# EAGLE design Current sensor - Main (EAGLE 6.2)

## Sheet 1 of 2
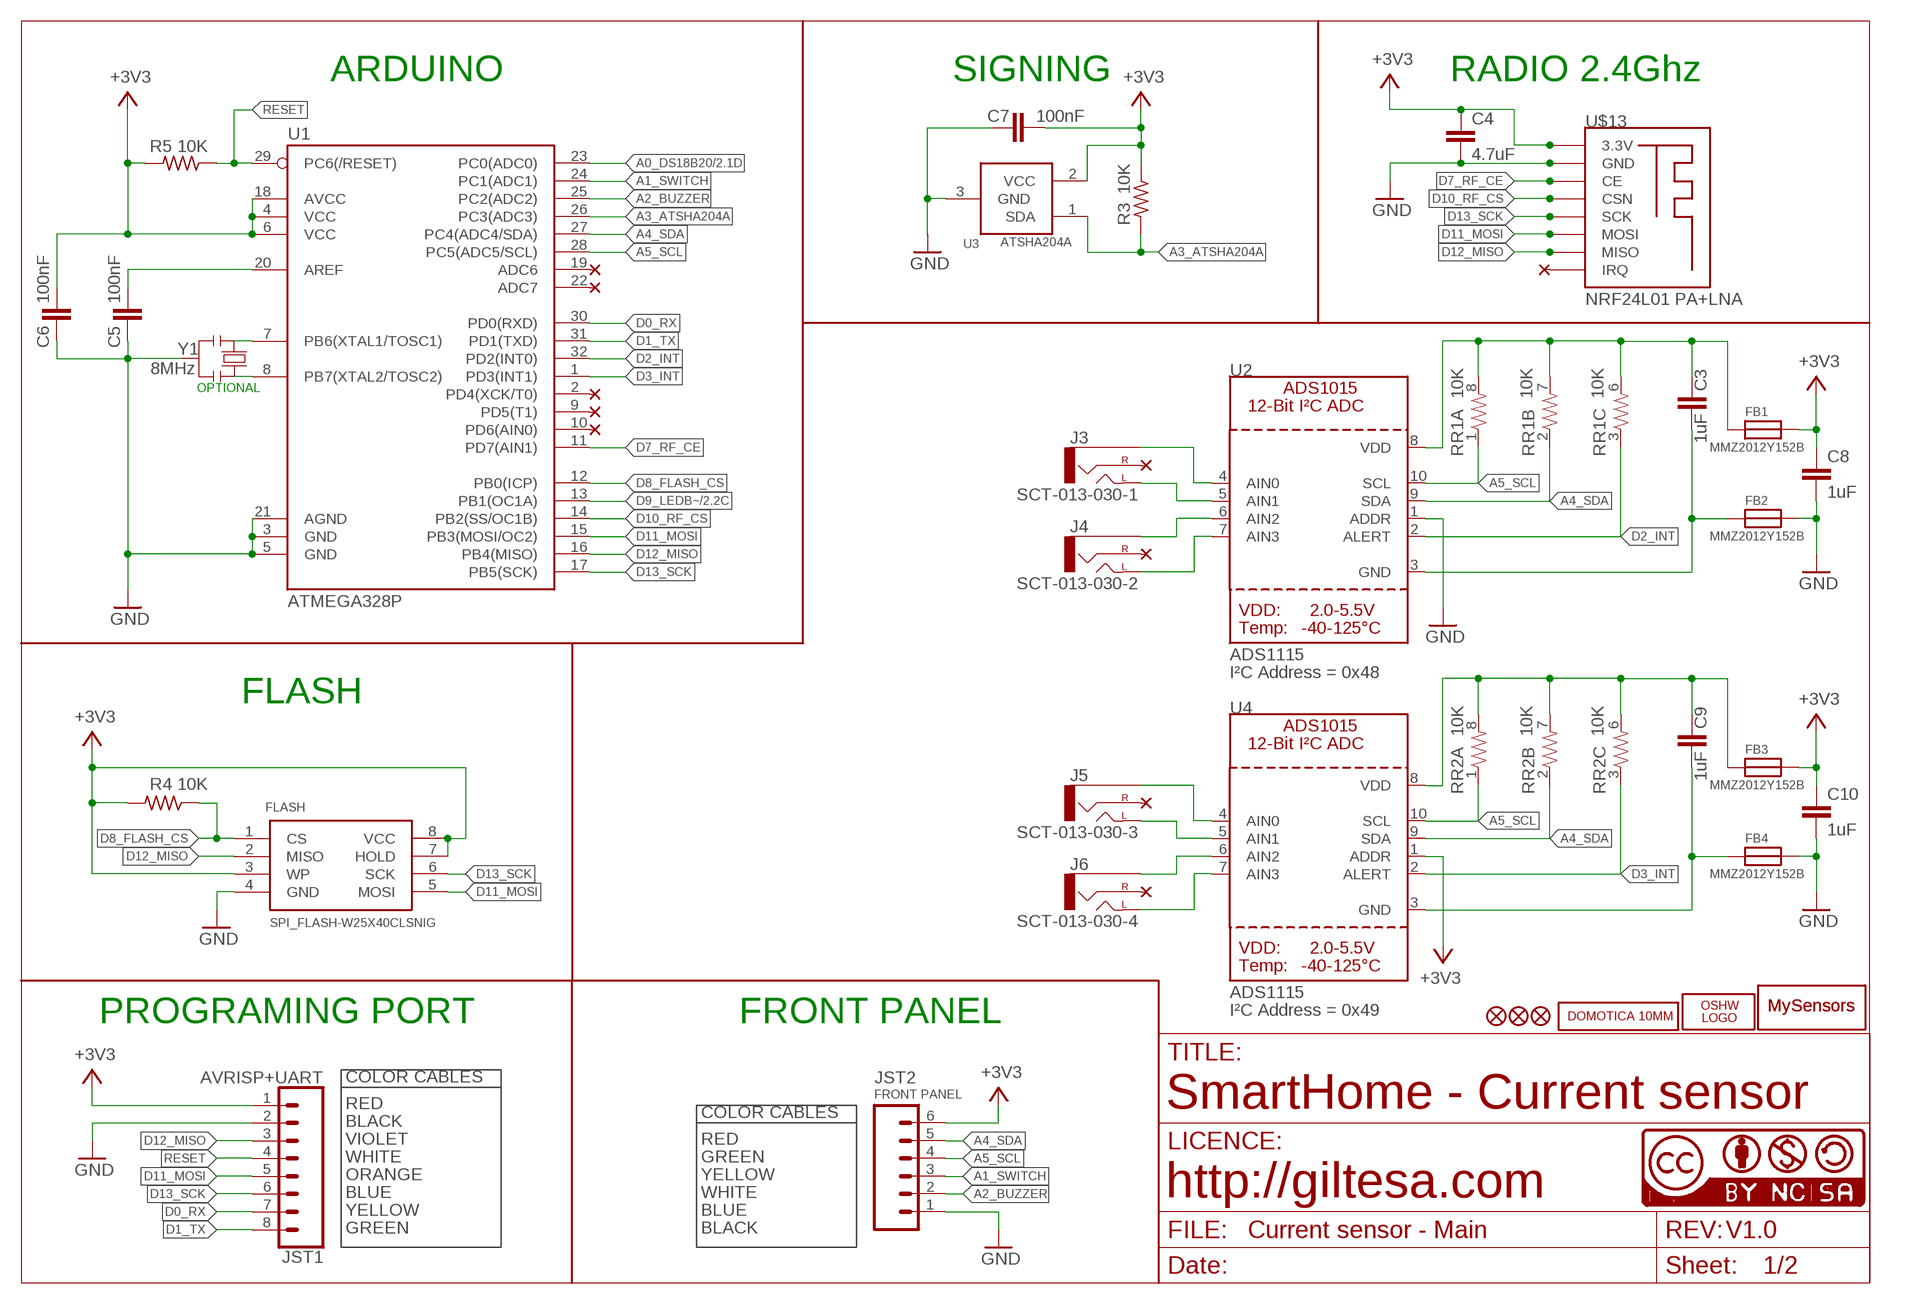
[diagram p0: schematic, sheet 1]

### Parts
C3  1uF  C0603  [C0603]
C4  4.7uF  C1206  [C1206]
C5  100nF  C0603  [C0603]
C6  100nF  C0603  [C0603]
C7  100nF  C0603  [C0603]
C8  1uF  C0603  [C0603]
C9  1uF  C0603  [C0603]
C10  1uF  C0603  [C0603]
FB1  MMZ2012Y152B  FERRITE0805  [0805]
FB2  MMZ2012Y152B  FERRITE0805  [0805]
FB3  MMZ2012Y152B  FERRITE0805  [0805]
FB4  MMZ2012Y152B  FERRITE0805  [0805]
FLASH  SPI_FLASH-W25X40CLSNIG  SPI_FLASH-X25XXSMD  [SO08]
J3  SCT-013-030-1  JACK_3.5MM  [JACK_3.5MM]
J4  SCT-013-030-2  JACK_3.5MM  [JACK_3.5MM]
J5  SCT-013-030-3  JACK_3.5MM  [JACK_3.5MM]
J6  SCT-013-030-4  JACK_3.5MM  [JACK_3.5MM]
JST1  AVRISP+UART  JST-8-1MM-SMD1  [JST-8-1MM-SMD]
JST2  FRONT PANEL  JST-6_1MM_SMD  [JST-6-1MM-SMD]
LOGO1  OSHW_LOGO_FILLX0150-NT  [OSHW_FILLX150_NOTEXT]
R3  10K  R0603  [R0603]
R4  10K  R0603  [R0603]
R5  10K  R0603  [R0603]
RR1  10K  RESISTOR-ARRAY0603-ARV  [0603-ARV]
RR2  10K  RESISTOR-ARRAY0603-ARV  [0603-ARV]
U1  ATMEGA328P  ATMEGA328P_TQFP  [TQFP32-08]
U2  ADS1115  ADC_ADS1015  [MSOP10]
U3  ATSHA204A  IC_ATSHA204A_CRYPT  [SOT23-3]
U4  ADS1115  ADC_ADS1015  [MSOP10]
U$2  MYSENSORS2  [MYSENSORS_20MM]
U$5  DOMOTICA-10MM  [DOMOTICA-10MM]
U$6  FIDUCIAL1X2  [FIDUCIAL-1X2]
U$7  FIDUCIAL1X2  [FIDUCIAL-1X2]
U$10  MYSENSORS4  [MYSENSORS_4MM]
U$13  NRF24L01 PA+LNA  NRF24L01SMD_RIGHT_IO2_B  [NRF24L01_SMD_RIGHT]
U$14  FIDUCIAL1X2  [FIDUCIAL-1X2]
U$20  CC-NC-BCNIX  [CC-NC-B_NIX]
Y1  8MHz  RESONATORMU  [RESONATOR]

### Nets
+3V3: C4.1 C6.2 C7.2 C8.1 C10.1 FB1.1 FB3.1 FLASH.3(WP) FLASH.7(HOLD) FLASH.8(VCC) JST1.1 JST2.6 R3.1 R4.2 R5.2 U1.4(VCC) U1.6(VCC) U1.18(AVCC) U3.2(VCC) U4.1(ADDR) U$13.B1(3.3V) ; also sheet 2
A0_DS18B20: U1.23(PC0(ADC0)) ; also sheet 2
A1_SWITCH: JST2.3 U1.24(PC1(ADC1))
A2_BUZZER: JST2.2 U1.25(PC2(ADC2))
A3_ATSHA204A: R3.2 U1.26(PC3(ADC3)) U3.1(SDA)
A4_SDA: JST2.5 RR1.2 RR2.2 U1.27(PC4(ADC4/SDA)) U2.9(SDA) U4.9(SDA)
A5_SCL: JST2.4 RR1.1 RR2.1 U1.28(PC5(ADC5/SCL)) U2.10(SCL) U4.10(SCL)
AIN0: J3.G U2.4(AIN0)
AIN1: J3.L U2.5(AIN1)
AIN2: J4.G U2.6(AIN2)
AIN3: J4.L U2.7(AIN3)
AIN4: J5.G U4.4(AIN0)
AIN5: J5.L U4.5(AIN1)
AIN6: J6.G U4.6(AIN2)
AIN7: J6.L U4.7(AIN3)
D0_RX: JST1.7 U1.30(PD0(RXD))
D1_TX: JST1.8 U1.31(PD1(TXD))
D2_INT: RR1.3 U1.32(PD2(INT0)) U2.2(ALERT)
D3_INT: RR2.3 U1.1(PD3(INT1)) U4.2(ALERT)
D7_RF_CE: U1.11(PD7(AIN1)) U$13.B2(CE)
D8_FLASH_CS: FLASH.1(CS) R4.1 U1.12(PB0(ICP))
D9_LEDB~: U1.13(PB1(OC1A)) ; also sheet 2
D10_RF_CS: U1.14(PB2(SS/OC1B)) U$13.B3(CSN)
D11_MOSI: FLASH.5(MOSI) JST1.5 U1.15(PB3(MOSI/OC2)) U$13.B5(MOSI)
D12_MISO: FLASH.2(MISO) JST1.3 U1.16(PB4(MISO)) U$13.B6(MISO)
D13_SCK: FLASH.6(SCK) JST1.6 U1.17(PB5(SCK)) U$13.B4(SCK)
GND: C4.2 C5.1 C6.1 C7.1 C8.2 C10.2 FB2.1 FB4.1 FLASH.4(GND) JST1.2 JST2.1 U1.3(GND) U1.5(GND) U1.21(AGND) U2.1(ADDR) U3.3(GND) U$13.B8(GND) Y1.2 ; also sheet 2
N$1: C9.2 FB3.2 RR2.6 RR2.7 RR2.8 U4.8(VDD)
N$2: C9.1 FB4.2 U4.3(GND)
N$3: C3.2 FB1.2 RR1.6 RR1.7 RR1.8 U2.8(VDD)
N$4: C3.1 FB2.2 U2.3(GND)
N$29: U1.7(PB6(XTAL1/TOSC1)) Y1.1
N$30: U1.8(PB7(XTAL2/TOSC2)) Y1.3
N$33: C5.2 U1.20(AREF)
RESET: JST1.4 R5.1 U1.29(PC6(/RESET))
Unconnected: J3.R J4.R J5.R J6.R RR1.4 RR1.5 RR2.4 RR2.5 U1.2(PD4(XCK/T0)) U1.9(PD5(T1)) U1.10(PD6(AIN0)) U1.19(ADC6) U1.22(ADC7) U$13.B7(IRQ)

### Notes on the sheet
- ARDUINO | SIGNING | RADIO 2.4Ghz
- OPTIONAL
- I²C Address = 0x48
- FLASH
- I²C Address = 0x49
- PROGRAMING PORT | FRONT PANEL
- COLOR CABLES
- RED | SmartHome - Current sensor
- COLOR CABLES
- BLACK
- VIOLET | RED
- WHITE | GREEN
- ORANGE | YELLOW
- BLUE | WHITE | http://giltesa.com
- YELLOW | BLUE
- GREEN | BLACK | V1.0

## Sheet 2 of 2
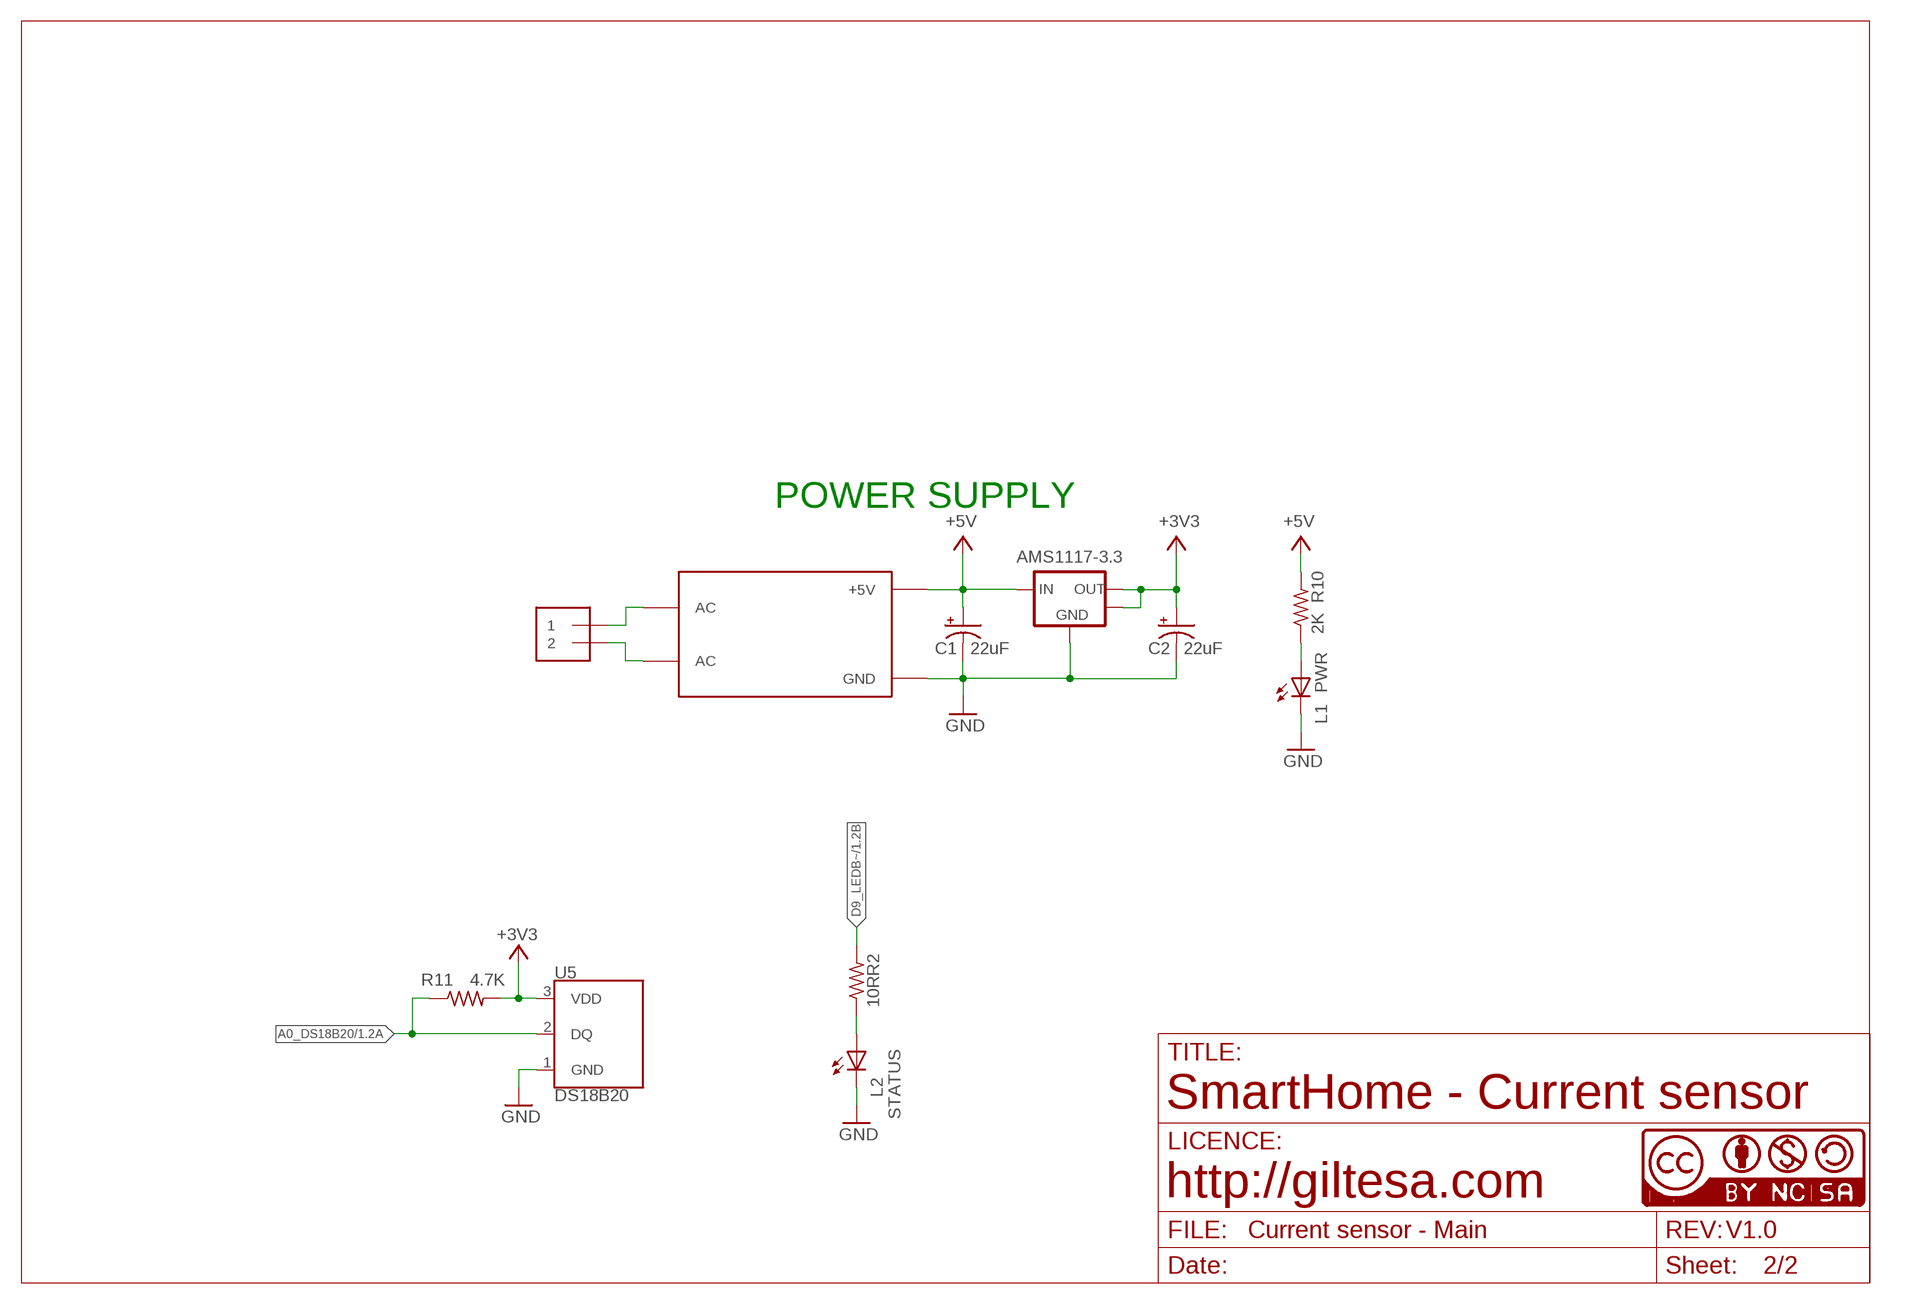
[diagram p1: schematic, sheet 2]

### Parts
AMS1117-3.3  AMS1117-3.3  AMS1117SOT89_2  [SOT89_2]
C1  22uF  CAP_POL3528  [EIA3528]
C2  22uF  CAP_POL3528  [EIA3528]
L1  PWR  LEDCHIP-LED0805  [CHIP-LED0805]
L2  STATUS  LEDCHIP-LED0805  [CHIP-LED0805]
R2  10R  R0603  [R0603]
R10  2K  R0603  [R0603]
R11  4.7K  R0603  [R0603]
U5  DS18B20  [DS18B20]
U$1  HILINK HLK-PM01 5V  HILINK_HLK-PM01_5V  [HILINK_HLK-PM01_5V]
U$12  230V  TERMINAL_15A_2PIN_RIGHT  [TERMINAL_15A_2PIN_RIGHT]
U$36  CC-NC-BCNIX  [CC-NC-B_NIX]

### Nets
+3V3: AMS1117-3.3.2(OUT) AMS1117-3.3.4(NC) C2.A(+) R11.2 U5.3(VDD) ; also sheet 1
+5V: AMS1117-3.3.3(IN) C1.A(+) R10.2 U$1.+5V
A0_DS18B20: R11.1 U5.2(DQ) ; also sheet 1
D9_LEDB~: R2.2 ; also sheet 1
GND: AMS1117-3.3.1(GND) C1.C(-) C2.C(-) L1.C L2.C U5.1(GND) U$1.GND ; also sheet 1
N$7: L2.A R2.1
N$8: L1.A R10.1
NEUTRAL: U$1.AC@2(AC) U$12.1
PHASE: U$1.AC@1(AC) U$12.2

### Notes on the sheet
- POWER SUPPLY
- SmartHome - Current sensor
- http://giltesa.com
- V1.0

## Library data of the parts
AMS1117-3.3 = ,giltesa:AMS1117
C1 C2 = SparkFun:CAP_POL: Capacitor Polarized
C3 C5-C10 = ,giltesa:C0603
C4 = ,giltesa:C1206
FB1-FB4 = microbuilder:FERRITE: Ferrite Bead
FLASH = SparkFun-DigitalIC:SPI_FLASH-X25XX: 8pin SPI Flash series x25xx. Works with devices like W25X32 and BR25L32
J3-J6 = ,giltesa:JACK_3.5MM
JST1 = ,giltesa:JST-8-1MM-SMD
JST2 = ,giltesa:JST-6
L1 L2 = led:LED: LED
LOGO1 = ohw-logo:OSHW_LOGO_FILL
R2-R5 R10 R11 = ,giltesa:R0603
RR1 RR2 = SparkFun-Passives:RESISTOR-ARRAY: Array Chip Resistor Source: RS Component / Phycomp
U1 = SparkFun-DigitalIC:ATMEGA328P_TQFP; PROD_ID: IC-09069; VALUE: ATMEGA328P_TQFP
U2 U4 = microbuilder:ADC_ADS1015: ADS1015 - 12-bit 4-Channel I2C ADC with Internal PGA VDD: 2.0-5.5V Sampling Rate: 3.3ksps Gain Settings: 2/3, 1, 2, 4, 8, 16 I2C Address: ADDR low = 1001000x, ADDR high = 1001001x Internal Comparator The ADS1015 includes an internal comparator that can be set to output a high-level on ALERT when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
U3 = TD-MySensors:IC_ATSHA204A_CRYPT
U5 = ,giltesa:DS18B20
U$1 = ,giltesa:HILINK_HLK-PM01_5V
U$2 U$10 = ,giltesa_logos:MYSENSORS
U$5 = ,giltesa_logos:DOMOTICA-10MM
U$6 U$7 U$14 = SparkFun:FIDUCIAL: Fiducial Alignment Points
U$12 = ,giltesa:TERMINAL_15A_2PIN_RIGHT
U$13 = ,giltesa:NRF24L01
U$20 U$36 = cc-by-nc-sa:CC-NC-BC: All hardware is licensed under the Creative Commons
Y1 = MySMD2:RESONATOR

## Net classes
2 gnd: width 0.305 mm, drill 0.406 mm, clearance 0.203 mm
3 usbvcc: width 0.203 mm, drill 0.406 mm, clearance 0.203 mm
4 USBpair: width 0.254 mm, drill 0.406 mm, clearance 0.61 mm

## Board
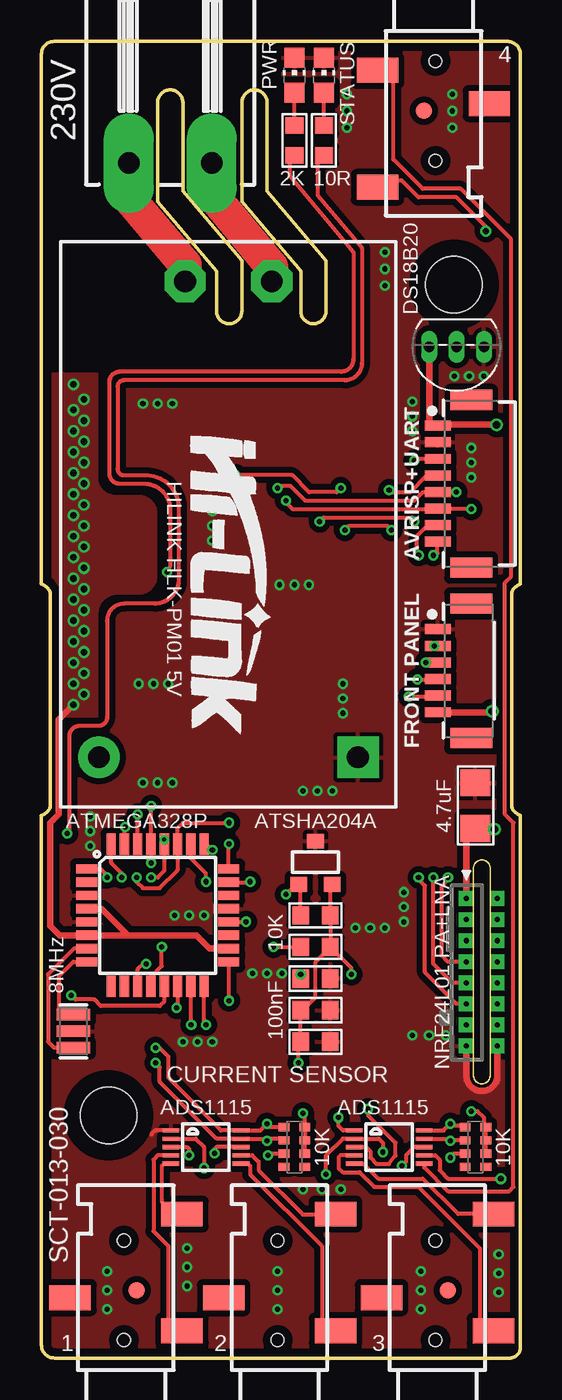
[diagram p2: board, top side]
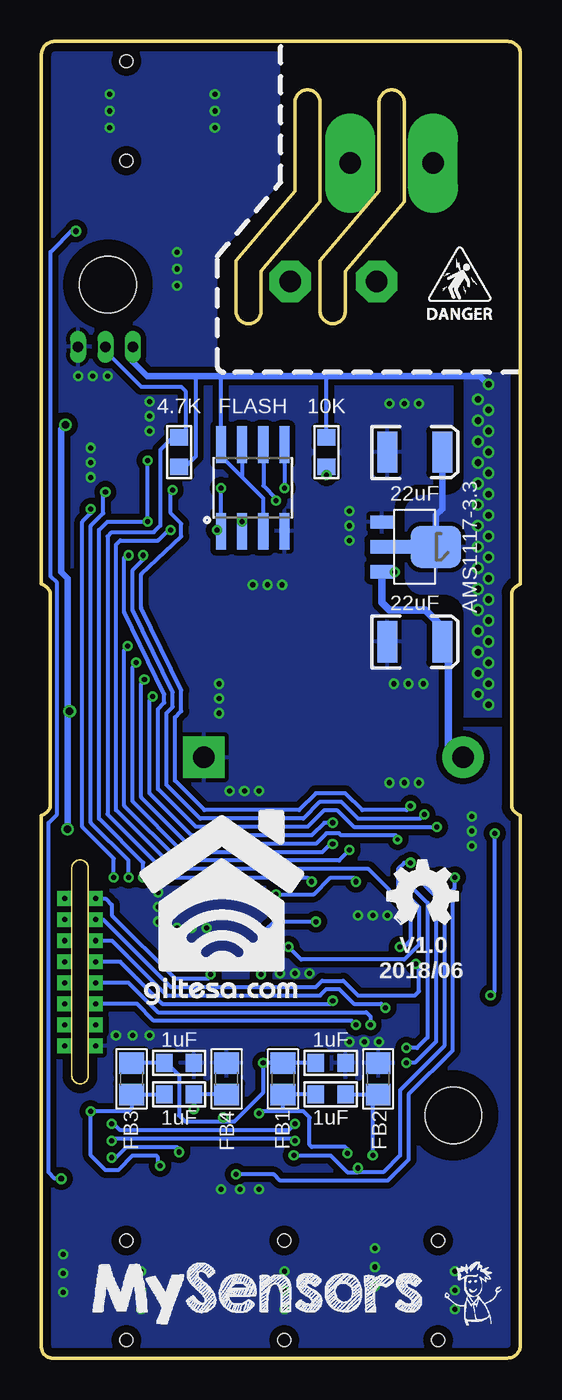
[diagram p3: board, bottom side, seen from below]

Size 28.91 x 79.4 mm. Coordinates in mm from the lower left corner, seen from the top.
Outline: 0.79,0 28.22,0 arc90 28.91,0.64 28.91,32.72 arc-50 28.37,33.22 28.37,46.18 arc-50 28.91,46.69 28.91,78.64 arc90 28.09,79.4 0.76,79.4 arc90 0,78.64 0,46.69 arc-50 0.53,46.18 0.53,33.22 arc-50 0,32.72 0,0.79 arc90 0.79,0
Outline: 7.01,75.72 arc-180 8.53,75.72 8.53,70.38 12.09,66.19 12.09,63.14 arc-180 10.57,63.14 10.57,65.56 7.01,69.75 7.01,75.72
Outline: 12.09,75.72 arc-180 13.61,75.72 13.61,70.38 17.17,66.19 17.17,63.14 arc-180 15.65,63.14 15.65,65.56 12.09,69.75 12.09,75.72
Copper layers (1*16): Top 0.035mm / dielectric 1.6mm / Bottom 0.035mm
Design rules: minimum track width 6mil, minimum drill 12mil, track to track 6mil, track to pad 6mil, pad to pad 6mil, via to via 8mil, smd to smd 0mil, copper to edge 20mil, drill to drill 10mil, minimum pad ring 6mil, minimum via ring 6mil, stop-mask expansion 0mil, vias tented up to drill 100mil, thermal gap 10mil
Holes 3.4 mm at 4.05,14.64 24.9,64.73
tRestrict: area 1.8,12.4 to 6.2,16.8; area 22.7,62.5 to 27.1,66.9; area 0,60 to 17.8,79.4; 14 lines
bRestrict: area 1.8,12.4 to 6.2,16.8; area 22.7,62.5 to 27.1,66.9; area 0,60 to 17.8,79.4; 14 lines

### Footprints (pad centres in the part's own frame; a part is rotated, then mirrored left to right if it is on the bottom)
SOT89_2 = smd 0.8 x 1.4: 1 -1.499,-1.981; 3 1.499,-1.981 | smd 0.8 x 2.54: 2 0,-1.409 | smd 2.54 x 3.048: 4 0,1.27
EIA3528 = smd 1.2 x 2.5: A 1.65,0; C -1.65,0
C0603 = smd 1 x 1.1: 1 -0.901,0; 2 0.901,0
C1206 = smd 1.6 x 1.8: 1 -1.362,0; 2 1.387,0
0805 = smd 1.3 x 1.5: 1 -0.95,0; 2 0.95,0
SO08 = smd 0.61 x 2.21: 1 -1.905,-2.616; 2 -0.635,-2.616; 3 0.635,-2.616; 4 1.905,-2.616; 5 1.905,2.616; 6 0.635,2.616; 7 -0.635,2.616; 8 -1.905,2.616
JACK_3.5MM = smd 2.5 x 1.5: G -3.5,2.446; L -3.5,-4.594; R 3.25,0.446 | hole 0.762: 0,3; 0,-3
JST-8-1MM-SMD = smd 0.6 x 1.55: 1 -3.5,-2.017; 2 -2.5,-2.017; 3 -1.5,-2.017; 4 -0.5,-2.017; 5 0.5,-2.017; 6 1.5,-2.017; 7 2.5,-2.017; 8 3.5,-2.017 | smd 1.219 x 2.54: NC1 -5.054,0; NC2 5.054,0
JST-6-1MM-SMD = smd 0.6 x 1.55: 1 -2.5,-2.017; 2 -1.5,-2.017; 3 -0.5,-2.017; 4 0.5,-2.017; 5 1.507,-2.017; 6 2.507,-2.017 | smd 1.219 x 2.54: P$7 -4.054,0; P$8 4.06,0
CHIP-LED0805 = smd 1.2 x 1.2: A 0,-1.05; C 0,1.05
R0603 = smd 1 x 1.1: 1 -0.901,0; 2 0.901,0
0603-ARV = smd 0.5 x 0.65: 1 -1.2,-0.625; 2 -0.4,-0.625; 3 0.4,-0.625; 4 1.2,-0.625; 5 1.2,0.625; 6 0.4,0.625; 7 -0.4,0.625; 8 -1.2,0.625
TQFP32-08 = smd 1.27 x 0.559: 1 -4.293,2.8; 2 -4.293,2; 3 -4.293,1.2; 4 -4.293,0.4; 5 -4.293,-0.4; 6 -4.293,-1.2; 7 -4.293,-2; 8 -4.293,-2.8; 17 4.293,-2.8; 18 4.293,-2; 19 4.293,-1.2; 20 4.293,-0.4; 21 4.293,0.4; 22 4.293,1.2; 23 4.293,2; 24 4.293,2.8 | smd 0.559 x 1.27: 9 -2.8,-4.293; 10 -2,-4.293; 11 -1.2,-4.293; 12 -0.4,-4.293; 13 0.4,-4.293; 14 1.2,-4.293; 15 2,-4.293; 16 2.8,-4.293; 25 2.8,4.293; 26 2,4.293; 27 1.2,4.293; 28 0.4,4.293; 29 -0.4,4.293; 30 -1.2,4.293; 31 -2,4.293; 32 -2.8,4.293
MSOP10 = smd 0.25 x 1: 1 -1,-2.113; 2 -0.5,-2.113; 3 0,-2.113; 4 0.5,-2.113; 5 1,-2.113; 6 1,2.113; 7 0.5,2.113; 8 0,2.113; 9 -0.5,2.113; 10 -1,2.113
SOT23-3 = smd 1 x 0.9: 1 -1,-1.3; 2 1,-1.3; 3 0,1.3
DS18B20 = drill 0.635 pad 0.864 long: 1 -1.651,0; 2 0,0; 3 1.651,0
HILINK_HLK-PM01_5V = drill 1.3 pad 2.5: +5V 31.109,2.3 | drill 1.3 pad 2.5 octagon: AC@1 2.409,12.73; AC@2 2.409,7.5 | drill 1.3 pad 2.5 square: GND 31.109,17.93
FIDUCIAL-1X2 = smd 1 x 1: 1 0,0
TERMINAL_15A_2PIN_RIGHT = drill 1.3 pad 3 long: 1 -2.5,-4.796; 2 2.5,-4.796
NRF24L01_SMD_RIGHT = drill 0.305 pad 0.889 square: B1 -4.445,-0.927; B2 -3.175,-0.927; B3 -1.905,-0.927; B4 -0.635,-0.927; B5 0.635,-0.927; B6 1.905,-0.927; B7 3.175,-0.927; B8 4.445,-0.927; T1 -4.445,0.927; T2 -3.175,0.927; T3 -1.905,0.927; T4 -0.635,0.927; T5 0.635,0.927; T6 1.905,0.927; T7 3.175,0.927; T8 4.445,0.927
RESONATOR = smd 0.7 x 2: 1 -1,0; 2 0,0; 3 1,0

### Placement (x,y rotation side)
AMS1117-3.3  6.38,48.92 270 bottom
C1  6.38,43.21 0 bottom
C2  6.38,54.64 0 bottom
C3  11.46,15.9 180 bottom
C4  26.19,33.3 90 top
C5  16.54,22.89 180 top
C6  16.54,20.98 180 top
C7  16.54,19.08 180 top
C8  11.46,17.81 0 bottom
C9  20.6,15.9 180 bottom
C10  20.6,17.81 0 bottom
FB1  14.33,16.84 270 bottom
FB2  8.59,16.84 270 bottom
FB3  23.47,16.84 270 bottom
FB4  17.73,16.84 270 bottom
FLASH  16.15,52.48 0 bottom
J3  4.98,4.09 180 top
J4  14.25,4.09 180 top
J5  23.77,4.09 180 top
J6  23.77,75.21 0 top
JST1  25.93,52.73 270 top
JST2  25.93,41.45 270 top
L1  15.27,77.37 0 top
L2  17.04,77.37 0 top
LOGO1  8.03,26.19 0 bottom
R2  17.04,73.43 270 top
R3  16.54,26.7 180 top
R4  11.71,54.64 90 bottom
R5  16.54,24.79 0 top
R10  15.27,73.43 270 top
R11  20.6,54.64 270 bottom
RR1  15.27,12.73 270 top
RR2  26.19,12.73 270 top
U1  7.01,26.7 0 top
U2  9.93,12.73 270 top
U3  16.54,29.87 0 top
U4  20.98,12.73 270 top
U5  25.04,60.99 180 top
U$1  1.17,67.34 270 top
U$2  25.81,2.06 0 bottom
U$5  23.01,21.23 0 bottom
U$6  5.74,4.09 0 top
U$7  24.54,4.09 0 top
U$10  4.85,1.8 0 bottom
U$12  7.77,76.86 0 top
U$13  26.57,23.27 270 top
U$14  23.08,75.21 0 top
U$16  [ELECTROCUTION_SMALL]  5.86,62.49 0 bottom
U$20  0.03,0.03 0 top
U$36  0.03,0.03 90 top
Y1  1.93,19.71 90 top

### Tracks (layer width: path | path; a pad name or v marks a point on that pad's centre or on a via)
+3V3  (via drill 0.3, 0.41, 0.46)
  Top 0.254: U3.2 17.44,28.47 R3.1 R5.2 | v15.52,17.81 15.52,18.96 C7.2 C6.2 15.77,20.98 16.54,21.74 16.54,23.89 R5.2 | U4.1 18.2,13.73 17.93,14 v17.93,14.5 | R5.2 17.44,24.78 18.69,23.52 v18.69,23.14
  Top 0.406: U$13.B1 25.64,31.29 C4.1 27.04,31.94 v27.33,31.9 | U1.18 10.15,24.7 9.35,25.5 5.23,25.5 | 5.23,25.5 U1.6 1.1,25.5 0.53,26.06 0.53,32.28 1.04,32.79 1.04,38.51 v1.93,39.4 | U1.4 3.63,27.1 5.23,25.5 | U5.3 23.39,56.29 23.45,56.23 JST1.1 23.97,56.29 v27.46,56.29 | JST2.6 27.14,38.95 v27.2,39.01
  Bottom 0.254: FB3.1 23.45,17.81 C10.1 21.36,17.81 20.6,17.04 20.6,14.63 20.22,14.25 17.93,14.25 | R4.2 11.71,59.1 11.84,59.22 | FLASH.3 15.52,51.84 16.85,53.18 | R11.2 20.23,53.73 19.58,54.38 19.58,59.22 | 16.85,53.18 18.06,54.38 FLASH.8 18.06,59.22 | FLASH.7 16.79,53.24 16.85,53.18 | C8.1 14.31,17.81 FB1.1 15.5,17.79 v15.52,17.81 15.52,16.03 17.3,14.25 17.93,14.25 | 17.93,14.25 v17.93,14.5 17.93,14.38 | U$13.B1 25.04,27.71 24.66,27.33 24.66,26.7 20.85,22.89 18.82,22.89 18.69,23.01 v18.69,23.14
  Bottom 0.406: C2.A 4.73,51.21 5.11,50.83 AMS1117-3.3.4 | v1.93,58.72 2.44,59.22 11.84,59.22 18.06,59.22 19.58,59.22 22.52,59.22 23.39,60.1 U5.3 | 27.33,38.89 27.33,47.02 27.71,47.4 27.71,56.03 v27.46,56.29 | v27.33,31.9 27.33,38.89 | 27.33,38.89 v27.2,39.01
  other vias: 1.93,40.67 1.93,41.94 1.93,43.21 1.93,44.48 1.93,45.75 1.93,47.02 1.93,48.29 1.93,49.56 1.93,50.83 1.93,52.1 1.93,53.37 1.93,54.64 1.93,55.91 1.93,57.18 2.57,57.81 2.57,56.54 2.57,55.27 2.57,54 2.57,52.73 2.57,51.46 2.57,50.19 2.57,48.92 2.57,47.65 2.57,46.38 2.57,45.11 2.57,43.84 2.57,42.57 2.57,41.3 2.57,40.03
  pour Bottom: 6.88,47.14 arc-90 5.87,46.13 4.6,46.13 arc90 3.33,44.86 3.33,38.63 0.79,38.63 0.79,45.87 arc50 0.28,46.38 0.28,59.35 3.33,59.35 3.33,52.98 arc90 4.6,51.97 5.87,51.97 arc-90 6.88,50.95
  pour Top: 6.88,47.14 arc-90 5.87,46.13 4.6,46.13 arc90 3.33,44.86 3.33,38.63 0.79,38.63 0.79,45.87 arc50 0.28,46.38 0.28,59.35 3.33,59.35 3.33,52.98 arc90 4.6,51.97 5.87,51.97 arc-90 6.88,50.95
+5V  (via drill 0.3)
  Top 0.254: v7.58,47.4 7.77,47.78 7.77,51.21 arc90 6.12,52.73 4.72,52.73 arc-90 4.09,53.37 4.09,58.84 arc-90 4.72,59.48 18.06,59.48 arc90 18.82,60.24 18.82,66.7 15.01,71.27 15.01,72.28 R10.2
  Bottom 0.254: v7.58,47.4 8.27,47.4 AMS1117-3.3.3
  Bottom 0.406: 4.72,44.09 C1.A
  Bottom 0.457: AMS1117-3.3.3 8.36,45.57 7.9,45.11 5.74,45.11 4.72,44.09 | U$1.+5V 3.84,36.23 4.34,36.73 4.34,42.82 C1.A
A0_DS18B20  (via drill 0.3)
  Top 0.254: U1.23 12.57,28.7 v12.6,28.73
  Bottom 0.254: U5.2 25.04,60.73 22.89,58.57 20.47,58.57 20.22,58.32 20.22,55.92 R11.1 20.97,55.54 21.74,54.76 21.74,50.19 22.12,49.81 24.66,49.81 24.92,49.56 24.92,32.79 21.11,28.98 12.85,28.98 v12.6,28.73
A1_SWITCH  (via drill 0.3)
  Top 0.254: U1.24 11.3,30.99 v11.33,31.01 | v23.2,41.94 23.9,41.94 JST2.3
  Bottom 0.254: v11.33,31.01 11.46,31.01 11.96,30.51 20.35,30.51 23.39,33.55 23.39,41.68 v23.2,41.94
A2_BUZZER  (via drill 0.3)
  Top 0.254: U1.25 9.96,30.99 v10.31,30.63 | v23.71,42.95 JST2.2
  Bottom 0.254: v10.31,30.63 10.95,30 20.6,30 23.9,33.3 23.9,42.7 v23.71,42.95
A3_ATSHA204A  (via drill 0.3)
  Top 0.254: v14.76,27.97 15.36,28.57 U3.1 15.63,28.47 R3.2 | v9.93,28.73 9.93,29.24 9.01,30.16 U1.26
  Bottom 0.254: v14.76,27.97 12.47,27.97 11.46,28.98 10.06,28.98 9.93,28.85 v9.93,28.73
A4_SDA  (via drill 0.3)
  Top 0.254: U4.9 24.67,13.23 v24.66,13.11 24.68,13.13 RR2.2 | RR1.2 14.64,13.22 14.63,13.23 13.74,13.23 v13.61,13.11 13.62,13.23 U2.9 10.57,13.23 7.14,16.66 7.14,17.55 v6.88,17.81 | v11.33,32.28 8.53,32.28 8.21,31.96 U1.27 8.21,29.42 7.14,28.35 6.12,28.35 5.74,28.73 v5.74,28.98 | v22.19,39.9 23.87,39.9 JST2.5
  Bottom 0.254: v13.61,13.11 13.74,13.23 24.54,13.23 v24.66,13.11 | v6.88,17.81 6.38,17.81 5.11,19.08 5.11,27.84 5.74,28.47 v5.74,28.98 | v11.33,32.28 11.84,32.28 12.6,31.52 19.84,31.52 22.38,34.06 22.38,39.65 v22.19,39.9
A5_SCL  (via drill 0.25, 0.3)
  Top 0.254: RR1.1 13.81,13.93 v13.61,14.12 13.22,13.73 U2.10 10.84,13.73 7.65,16.92 7.65,18.19 7.14,18.69 v6.88,18.69 | U4.10 24.27,13.73 v24.66,14.12 24.79,14 25.3,14 25.37,13.93 RR2.1 | v6.63,28.98 7.01,28.98 7.41,29.38 U1.28 7.41,31.25 v7.41,31.27 | v22.69,40.92 23.88,40.92 JST2.4
  Bottom 0.254: v13.61,14.12 14,13.74 24.16,13.74 24.54,14.12 v24.66,14.12 | v6.88,18.69 6.25,18.69 5.61,19.33 5.61,27.46 6.63,28.47 v6.63,28.98 | v7.41,31.27 7.39,31.39 7.52,31.52 10.82,31.52 10.95,31.65 11.71,31.65 12.34,31.01 20.09,31.01 22.89,33.81 22.89,40.67 v22.69,40.92
AIN0
  Top 0.254: U2.4 7.02,12.23 6.76,11.96 6.76,7.65 7.65,6.76 7.65,2.06 7.9,1.8 8.32,1.8 J3.G
AIN1
  Top 0.254: U2.5 7.41,11.73 7.26,11.58 7.26,9.42 7.52,9.17 7.99,9.17 J3.L
AIN2
  Top 0.254: J4.G 17.59,1.8 17.3,1.8 16.92,2.18 16.92,6.76 12.6,11.07 12.6,11.58 12.46,11.73 U2.6
AIN3
  Top 0.254: J4.L 17.73,8.66 15.77,8.66 13.11,11.33 13.11,11.84 12.72,12.23 U2.7
AIN4
  Top 0.254: J5.G 27.24,1.68 26.57,1.68 26.44,1.8 26.44,6.63 22.76,10.31 20.09,10.31 19.2,11.2 18.19,11.2 17.93,11.46 17.93,12.09 18.07,12.23 U4.4
AIN5
  Top 0.254: U4.5 19.44,11.73 20.35,10.82 23.01,10.82 25.15,8.68 J5.L 26.92,9.04
AIN6
  Top 0.254: U4.6 23.09,11.5 24.54,10.06 28.22,10.06 28.47,10.31 28.47,32.28 27.97,32.79 27.97,46.76 28.35,47.14 28.35,67.46 25.3,70.51 23.01,70.51 21.23,72.29 21.23,77.5 20.98,77.75 20.37,77.75 J6.G
AIN7  (via drill 0.36)
  Top 0.254: U4.7 23.77,12.23 24.03,11.96 24.03,11.33 24.54,10.82 v27.71,10.82 | v26.82,67.97 26.95,68.1 25.04,70 22.76,70 21.74,71.02 20.68,71.02 J6.L 20.76,70.13
  Bottom 0.254: v27.71,10.82 28.09,10.82 28.47,11.2 28.47,32.28 27.97,32.79 27.97,46.76 28.35,47.14 28.35,66.7 26.95,68.1 v26.82,67.97
D0_RX  (via drill 0.3)
  Top 0.254: U1.30 5.81,32.73 v5.8,32.79 | JST1.7 23.43,50.23 23.27,50.06 23.14,50.06 22.63,49.56 22.63,48.54 v22.76,48.41
  Bottom 0.254: v5.8,32.79 6.06,32.54 9.8,32.54 10.82,33.55 12.09,33.55 13.11,32.54 19.33,32.54 21.36,34.57 21.36,38.89 20.98,39.27 20.98,40.16 23.39,45.11 23.39,47.52 22.76,48.16 v22.76,48.41
D1_TX  (via drill 0.3)
  Top 0.254: U1.31 5.01,31.93 v5.04,32.03 | v23.65,48.41 23.77,48.41 23.9,48.54 23.9,49.22 JST1.8
  Bottom 0.254: v5.04,32.03 10.06,32.03 11.07,33.05 11.84,33.05 12.85,32.03 19.58,32.03 21.87,34.32 21.87,39.14 21.49,39.52 21.49,40.03 23.9,44.98 23.9,48.29 23.77,48.41 v23.65,48.41
D2_INT  (via drill 0.3)
  Top 0.254: RR1.3 13.91,12.33 v13.68,12.22 | U2.2 9.3,13.23 9.8,12.73 v9.8,11.46 | v4.85,28.98 4.85,29.24 4.22,29.87 U1.32
  Bottom 0.254: v13.68,12.22 11.46,12.22 10.44,11.2 9.8,11.2 | v4.85,28.98 4.85,28.47 4.6,28.22 4.6,18.82 7.26,16.15 7.26,12.22 8.28,11.2 9.8,11.2 | 9.8,11.2 v9.8,11.46
D3_INT  (via drill 0.3)
  Top 0.254: RR2.3 24.9,12.33 v24.66,12.09 | v20.6,12.42 20.6,12.98 20.35,13.23 U4.2 18.18,13.23 17.17,12.22 v17.17,11.07 | U1.1 3.58,29.5 3.96,29.11 v3.96,28.98
  Bottom 0.254: v24.66,12.09 24.41,12.09 23.77,12.73 20.73,12.73 v20.6,12.42 | v17.17,11.07 14.88,11.07 14.5,10.69 8.03,10.69 6.76,11.96 6.76,15.9 4.09,18.57 4.09,28.22 3.96,28.35 v3.96,28.98
D7_RF_CE  (via drill 0.3)
  Top 0.254: v6.31,23.77 6.12,23.77 5.81,23.46 U1.11
  Bottom 0.254: U$13.B2 25.17,26.44 21.11,22.38 12.34,22.38 11.96,22.76 10.69,22.76 9.8,21.87 6.38,21.87 6.12,22.12 6.12,23.65 v6.31,23.77
D8_FLASH_CS  (via drill 0.3)
  Top 0.254: v18.06,52.48 17.81,52.22 16.15,52.22 15.14,53.24 v11.71,53.24 | U1.12 6.61,22.99 7.26,23.65 v7.26,24.79 | v18.31,49.94 18.57,50.19 20.85,50.19 v21.11,49.94
  Bottom 0.254: v18.06,52.48 FLASH.1 18.14,49.94 v18.31,49.94 | v11.71,53.24 R4.1 | v7.26,24.79 7.01,24.79 6.63,25.17 6.63,26.95 9.17,29.49 20.85,29.49 24.41,33.05 24.41,49.05 24.16,49.3 21.87,49.3 21.23,49.94 v21.11,49.94
D9_LEDB~  (via drill 0.3)
  Top 0.254: R2.2 17.03,72.53 16.66,72.16 16.66,70.13 19.33,66.95 19.33,59.99 arc-90 18.31,58.97 4.98,58.97 arc90 4.6,58.59 4.6,53.62 arc90 4.98,53.24 6.25,53.24 arc-90 8.28,51.33 8.28,47.02 arc-90 6.88,45.49 4.98,45.49 arc90 3.96,44.48 3.96,38.63 arc-90 3.45,38.13 2.31,38.13 arc90 1.68,37.49 1.68,31.78 v1.55,31.65 | U1.13 7.39,22.38 7.39,21.49 7.14,21.23 3.58,21.23 3.2,21.62 2.06,21.62 v1.8,21.87
  Bottom 0.254: v1.55,31.65 1.55,22.12 v1.8,21.87
D10_RF_CS  (via drill 0.3)
  Top 0.254: U1.14 8.21,21.16 v8.15,21.11
  Bottom 0.254: U$13.B3 24.66,25.17 21.36,21.87 12.09,21.87 11.71,22.25 10.95,22.25 10.06,21.36 8.41,21.36 v8.15,21.11
D11_MOSI  (via drill 0.3)
  Top 0.254: v14.25,52.48 14.38,52.6 15.01,52.6 15.9,51.71 22.5,51.71 23.01,52.22 JST1.5 | v9.04,20.09 9.04,22.37 U1.15 | U$13.B5 24.79,22.63 23.65,23.77 v23.65,28.98 | JST1.5 24.15,52.23 24.16,52.22 | v25.04,52.22 JST1.5
  Bottom 0.254: FLASH.5 v14.25,52.48 | v9.04,20.09 9.04,20.6 9.3,20.85 21.87,20.85 23.65,22.63 U$13.B5 | v23.65,28.98 23.65,30 25.93,32.28 25.93,50.19 25.17,50.95 25.17,52.1 v25.04,52.22
D12_MISO  (via drill 0.3)
  Top 0.254: v16.79,50.44 17.04,50.7 22.38,50.7 22.5,50.57 v22.5,50.44 | v22.5,54.13 22.63,54.25 23.89,54.25 JST1.3 | v9.93,20.09 9.8,20.22 U1.16 | U$13.B6 25.04,21.36 23.14,23.27 23.14,28.47 22.76,28.85 v22.76,28.98
  Bottom 0.254: FLASH.2 v16.79,50.44 | v22.5,54.13 v22.5,50.44 24.92,50.44 25.43,49.94 25.43,32.54 22.76,29.87 v22.76,28.98 | v9.93,20.09 10.19,20.35 22.12,20.35 23.14,21.36 U$13.B6
D13_SCK  (via drill 0.3)
  Top 0.254: v14.76,51.71 14.76,51.59 15.14,51.21 23.89,51.21 JST1.6 23.94,51.21 v25.93,51.21 | v11.33,21.55 11.33,23.87 U1.17 | U$13.B4 24.54,23.9 24.16,24.28 24.16,28.47 24.54,28.85 v24.54,28.98
  Bottom 0.254: FLASH.6 15.52,52.6 14.76,51.84 v14.76,51.71 | v11.33,21.55 11.33,21.49 11.46,21.36 21.62,21.36 24.16,23.9 U$13.B4 | v24.54,28.98 24.54,30.12 26.44,32.03 26.44,50.44 25.93,50.95 v25.93,51.21
GND  (via drill 0.3)
  Top 0.254: U2.1 6.87,13.73 6.63,13.49
  Top 0.406: U$13.B8 25.64,17.04 arc180 27.52,17.04 27.52,18.82
  other vias: 14.25,4.09 14.25,2.95 14.25,5.23 22.89,4.09 22.89,5.23 22.89,2.95 27.58,5.11 27.58,3.96 27.58,6.25 8.79,6.63 8.79,5.49 8.79,4.34 15.77,10.19 16.92,10.19 18.06,10.19 3.96,4.09 3.96,5.23 3.96,2.95 24.79,75.21 24.79,76.23 24.79,74.19 18.44,76.23 18.44,75.21 18.44,74.19 20.73,65.68 20.73,64.67 20.73,66.7 22.38,19.46 24.41,19.46 23.39,19.46 8.53,19.08 9.42,19.08 10.31,19.08 18.95,25.93 19.84,25.93 20.73,25.93 8.03,26.7 8.92,26.7 9.8,26.7 12.73,23.2 13.61,23.2 14.5,23.2 21.87,28.09 21.87,27.2 21.87,26.31 6.12,34.7 7.01,34.7 7.9,34.7 2.95,30.89 2.95,31.78 2.95,32.66 15.77,34.19 16.66,34.19 17.55,34.19 18.19,38.89 18.19,39.78 18.19,40.67 5.87,40.67 6.76,40.67 7.65,40.67 10.31,51.08 10.31,50.19 10.31,49.3 14.38,46.63 15.27,46.63 16.15,46.63 6.12,57.56 7.01,57.56 7.9,57.56 24.92,59.21 25.81,59.21 26.7,59.21 22.38,57.68 22.38,56.79 22.38,55.91 25.93,54.89 25.93,54 25.93,53.11
  pour Top (isolate 0.356): -0.61,-0.61 29.24,-0.61 29.24,80.04 -0.61,80.04
  pour Bottom (isolate 0.356): -0.61,-0.61 29.24,-0.61 29.24,80.04 -0.61,80.04
N$1  (via drill 0.3)
  Top 0.254: RR2.6 RR2.7 RR2.8 26.7,13.94 26.7,14.5 26.31,14.88 v25.93,14.88 | U4.8 22.5,12.73 22,12.22 22,11.84 v21.74,11.58
  Bottom 0.254: 21.79,15.76 C9.2 21.51,15.89 FB3.2 23.47,15.06 23.65,14.88 v25.93,14.88 25.93,12.22 25.04,11.33 24.28,11.33 23.39,12.22 22,12.22 21.87,12.09 21.87,11.71 v21.74,11.58
N$2  (via drill 0.3)
  Top 0.254: U4.3 19.58,12.73 19.84,12.47 19.84,12.09 20.22,11.71 20.98,11.71 21.36,12.22 21.36,12.98 19.71,14.63 v19.71,15.01
  Bottom 0.254: FB4.2 19.7,15.89 C9.1 v19.7,15.02 v19.71,15.01
N$3  (via drill 0.3)
  Top 0.254: RR1.6 RR1.7 RR1.8 15.9,14.63 v15.77,14.76 | U2.8 10.57,12.73 10.44,12.6 v10.44,12.34
  Bottom 0.254: FB1.2 14.51,15.76 | C3.2 14.32,15.9 FB1.2 | v10.44,12.34 10.44,12.6 10.57,12.73 12.6,12.73 12.73,12.85 12.73,14.5 13.11,14.88 14.33,14.88 | 14.33,14.88 15.65,14.88 v15.77,14.76 | 14.33,14.88 FB1.2
N$4  (via drill 0.3)
  Top 0.254: U2.3 8.79,12.73 8.92,12.6 v8.92,12.22
  Bottom 0.254: 8.66,15.56 FB2.2 | C3.1 8.6,15.9 FB2.2 | v8.92,12.22 8.92,15.56 FB2.2
N$7
  Top 0.254: R2.1 L2.A
N$8
  Top 0.254: 15.25,76.31 L1.A R10.1
N$29
  Top 0.254: U1.7 1.96,24.7 0.41,23.14 0.41,19.08 0.77,18.71 Y1.1
N$30
  Top 0.254: Y1.3 1.31,20.71 1.07,20.98 1.07,23.04 1.93,23.9 U1.8
N$33  (via drill 0.3)
  Top 0.254: U1.20 12.33,26.3 v12.34,26.31 | v15.65,23.14 15.65,22.9 C5.2
  Bottom 0.254: v12.34,26.31 14.88,26.31 15.39,25.81 15.39,23.39 v15.65,23.14
NEUTRAL
  Top 2.032: U$1.AC@2 8.66,65.94 5.23,70 U$12.1
PHASE
  Top 2.032: U$1.AC@1 13.87,65.81 10.31,70.13 U$12.2
RESET  (via drill 0.3)
  Top 0.254: v6.63,29.87 6.61,30.02 U1.29 6.61,33.28 v6.63,33.3 | v14,24.79 R5.1 | v20.98,52.35 21.11,52.22 22.25,52.22 23.27,53.24 23.91,53.24 JST1.4
  Bottom 0.254: v6.63,29.87 7.01,29.87 7.39,29.49 7.39,28.47 6.12,27.2 6.12,24.92 7.01,24.03 13.23,24.03 v14,24.79 | v6.63,33.3 6.88,33.05 9.55,33.05 10.57,34.06 12.34,34.06 13.36,33.05 19.08,33.05 20.85,34.82 20.85,38.63 20.47,39.01 20.47,40.28 22.89,45.24 22.89,47.27 20.47,49.56 20.47,50.32 21.11,50.95 21.11,52.22 v20.98,52.35

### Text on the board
tPlace: 4 | CURRENT SENSOR | SCT-013-030 | 1 | 2 | 3
bPlace: V1.0 | 2018/06

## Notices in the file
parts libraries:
SparkFun-DigitalIC: Licensing: Creative Commons ShareAlike 4.0 International - https://creativecommons.org/licenses/by-sa/4.0
SparkFun-Aesthetics: Licensing: CC v3.0 Share-Alike You are welcome to use this library for commercial purposes.
